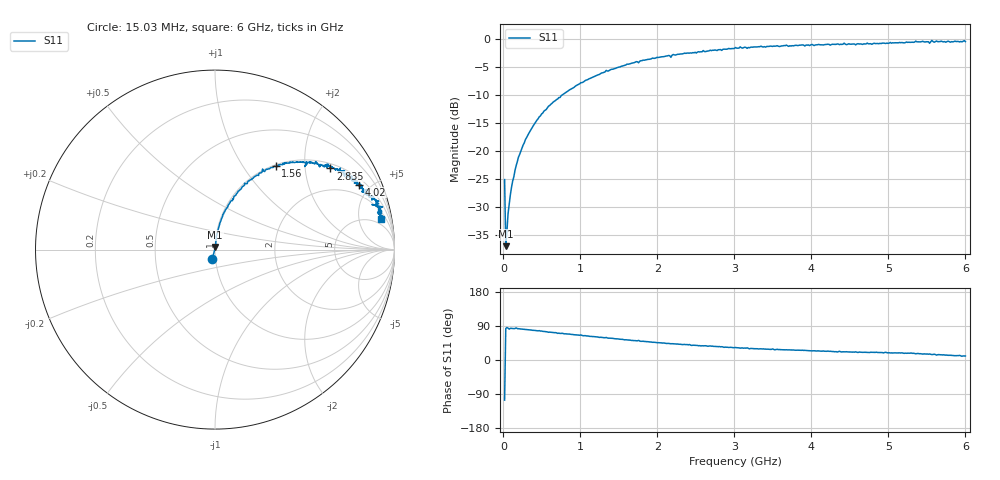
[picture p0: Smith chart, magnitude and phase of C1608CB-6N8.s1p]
!	Network	Analyzer	HP8753E.07.74:	Oct	30	2002	Serial	No.	JP38451487
!	Hewlett-Packard
!	7	Sep	2009	9:32:18
!	Frequency	S11
#	HZ	S	RI	R	50
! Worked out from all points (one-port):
!   400 points, 15.03 MHz to 6 GHz, reference 50 ohm
!   lowest |S11| = -37.0 dB at 30.03 MHz (marker M1), VSWR 1.03, Z = 50.1 + j1.4 ohm
!   |S11| at or under -10 dB: start of sweep to 767.7 MHz
!   S11 on the Smith chart (normalised r, x): 15.03 MHz: 0.96, -0.10; 1.56 GHz: 1.03, +1.42; 2.835 GHz: 1.15, +2.72; 4.02 GHz: 1.33, +4.25; 6 GHz: 3, +10
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1.502992e7  -0.0152 -0.0532
3.002985e7  0.00169 0.014
6.00297e7  0.00286 0.0274
9.002955e7  0.00445 0.0404
1.200294e8  0.00625 0.0535
1.95029e8  0.0112 0.0871
2.850286e8  0.0205 0.124
4.650277e8  0.0435 0.196
7.650262e8  0.106 0.297
1.335023e9  0.265 0.449
1.515022e9  0.323 0.457
1.560022e9  0.338 0.464
2.265019e9  0.538 0.488
2.595017e9  0.623 0.475
2.835016e9  0.643 0.452
3.015015e9  0.699 0.454
3.195014e9  0.722 0.408
3.765011e9  0.772 0.384
4.02001e9  0.802 0.362
4.515007e9  0.833 0.32
5.265004e9  0.885 0.285
5.445003e9  0.912 0.255
5.520002e9  0.905 0.247
5.535002e9  0.874 0.251
5.565002e9  0.934 0.238
5.595002e9  0.896 0.245
5.625002e9  0.929 0.213
6e9  0.926 0.172
